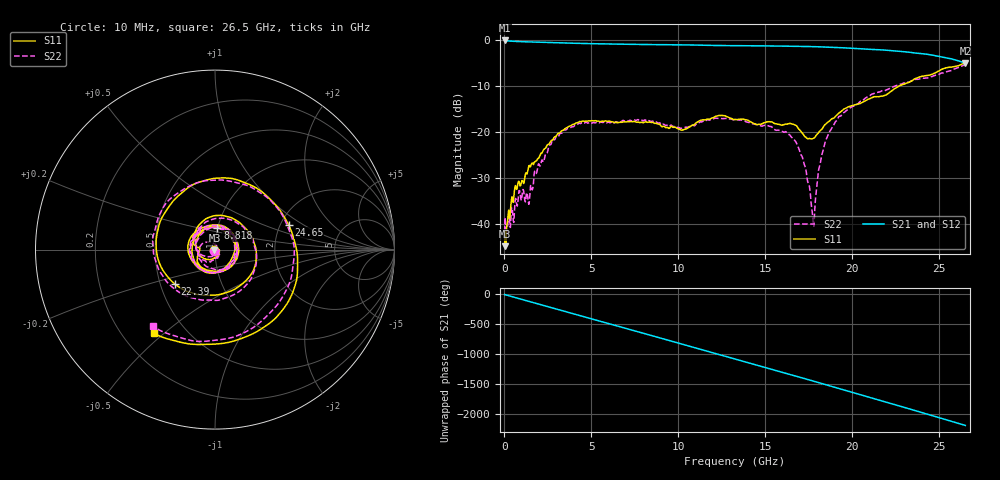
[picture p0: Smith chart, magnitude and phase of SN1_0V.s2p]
!Agilent Technologies,N5222A,MY51421700,A.10.00.00
!Agilent N5222A: A.10.00.00
!Date: Thursday, April 02, 2015 22:47:43
!Correction: S11(Full 2 Port(1,2))
!S21(Full 2 Port(1,2))
!S12(Full 2 Port(1,2))
!S22(Full 2 Port(1,2))
!S2P File: Measurements: S11, S21, S12, S22:
# Hz S  dB  R 50
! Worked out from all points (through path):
!   801 points, 10 MHz to 26.5 GHz, reference 50 ohm
!   highest |S21| = 0.00 dB at 10 MHz (marker M1); lowest = -4.9 dB at 26.5 GHz (marker M2)
!   group delay of S21, straight-line fit = 228 ps
!   lowest |S11| = -44.8 dB at 10 MHz (marker M3), VSWR 1.01, Z = 49.7 - j0.484 ohm
!   |S11| at or under -10 dB: start of sweep to 22.65 GHz
!   |S22| runs from -43.1 to -5.2 dB; largest |S21 - S12| = 0.0024
!   S11 on the Smith chart (normalised r, x): 10 MHz: 0.99, -0.01; 8.818 GHz: 1.00, +0.25; 22.39 GHz: 0.59, -0.25; 24.65 GHz: 2.22, +0.75; 26.5 GHz: 0.33, -0.46
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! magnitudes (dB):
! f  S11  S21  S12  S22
! 10 MHz  -44.8  0.0  0.0  -41.7
! 705.4 MHz  -32.5  -0.2  -0.2  -35.7
! 1.335 GHz  -28.5  -0.3  -0.3  -33.9
! 1.831 GHz  -26.2  -0.4  -0.4  -29.0
! 2.858 GHz  -21.1  -0.5  -0.5  -21.7
! 4.447 GHz  -17.6  -0.7  -0.7  -17.9
! 8.818 GHz  -18.2  -0.9  -0.9  -18.0
! 8.851 GHz  -18.3  -0.9  -0.9  -18.0
! 10.24 GHz  -19.5  -1.0  -1.0  -19.1
! 12.26 GHz  -16.4  -1.1  -1.1  -17.0
! 13.26 GHz  -17.2  -1.1  -1.1  -17.3
! 16.63 GHz  -18.3  -1.3  -1.3  -21.5
! 17.23 GHz  -20.8  -1.3  -1.3  -26.9
! 17.69 GHz  -21.4  -1.4  -1.4  -37.3
! 17.82 GHz  -21.2  -1.4  -1.4  -38.2
! 18.09 GHz  -19.9  -1.4  -1.4  -27.8
! 18.35 GHz  -18.7  -1.4  -1.4  -23.4
! 19.08 GHz  -16.3  -1.5  -1.5  -17.5
! 22.1 GHz  -11.5  -2.2  -2.2  -10.6
! 22.39 GHz  -10.6  -2.3  -2.3  -10.0
! 24.65 GHz  -7.3  -3.2  -3.2  -7.8
! 26.5 GHz  -4.8  -4.9  -4.9  -5.2
